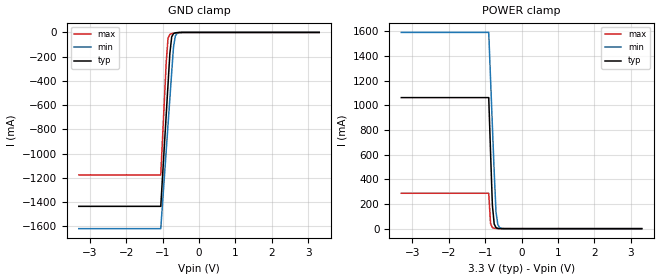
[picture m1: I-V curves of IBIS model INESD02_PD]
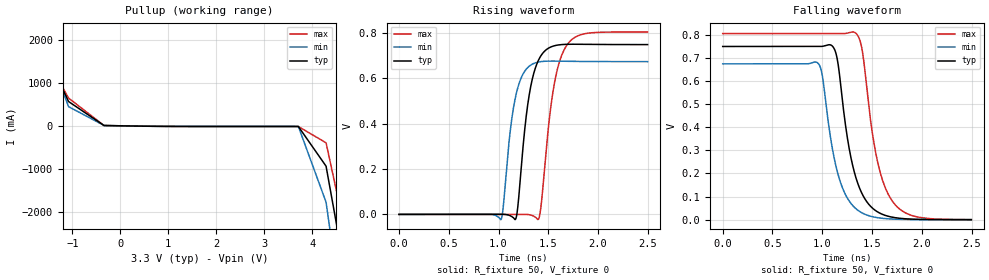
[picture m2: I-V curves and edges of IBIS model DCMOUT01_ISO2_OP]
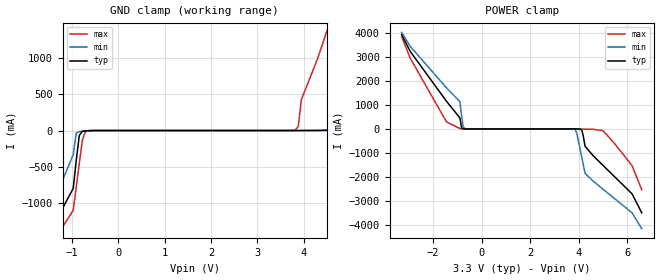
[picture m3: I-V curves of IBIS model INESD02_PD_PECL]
|   This file is an IBIS representation of the   |
|   Integrated Device Technology, Inc.   |
|   ICS841608I   |
|   FEMTOCLOCKS CRYSTAL-TO-HCSL CLOCK GENERATOR   |
[IBIS Ver]   4.1
[File name]   841608i_3v3.ibs
[File Rev]   1.0
[Date]   5 Mar 2010
[Source]   Originated at Integrated Device Technology, Inc.
[Disclaimer]
IDT hereby grants the user of this IBIS model a non-exclusive,
nontransferable license to use this IBIS model under the following terms.
Before using this IBIS model, the user should read this license.
If the user does not accept these terms,  the IBIS model should be
returned to IDT within 30 days.
   The user is granted this license only to use the IBIS model and
is not granted rights to sell, load, rent, lease or license the IBIS
model in whole or in part, or in modified form to anyone other than
user. User may modify the IBIS model to suit its specific
applications but rights to derivative works and such modifications
shall belong to IDT.
   This IBIS model is provided on an "AS IS" basis and IDT makes
absolutely no warranty with respect to the information contained
herein. IDT DISCLAIMS AND CUSTOMER WAIVES ALL WARRANTIES, EXPRESS
OR IMPLIED, INCLUDING WARRANTIES OF MERCHANTABILITY OR FITNESS FOR
A PARTICULAR PURPOSE. The entire risk as to quality and performance
is with the Customer. ACCORDINGLY, IN NO EVENT SHALL THE COMPANY BE
LIABLE FOR ANY DAMAGES, WHETHER IN CONTRACT OR TORT,INCLUDING ANY
LOST PROFITS OR OTHER INCIDENTAL, CONSEQUENTIAL, EXEMPLARY, OR
PUNITIVE DAMAGES ARISING OUT OF THE USE OR APPLICATION OF THE IBIS
model provided in this package. Further, IDT reserves the right to
make changes without notice to any product herein to improve
reliability, function, or design. IDT does not convey any license
under patent rights or any other intellectual property rights,
including those of third parties.
   IDT is not obligated to provide maintenance or support
for the licensed IBIS model.
[Copyright]   Copyright 2008 by Integrated Device Technology, Inc.
[Component]   ICS841608KI
[Manufacturer] Integrated Device Technology, Inc.
[Package]
|LD QFN 32
|lead + wire   typ   min   max
R_pkg   72.4655m   58.886m   86.045m
L_pkg   1.47175nH   1.11650nH   1.77850nH
C_pkg   0.07747pF   0.07444pF   0.08050pF
[Pin] signal_name   model_name   R_pin   L_pin   C_pin
1   XTAL_IN  NC   86.045m   1.77850nH   0.08050pF
2   XTAL_OUT NC   76.996m   1.55783nH   0.07848pF
3   MR/nOE   INESD02_PD   67.941m   1.33717nH   0.07646pF
4   VDD   POWER   58.886m   1.11650nH   0.07444pF
5   Q0   DCMOUT01_ISO2_OP   58.886m   1.11650nH   0.07444pF
6   nQ0   DCMOUT01_ISO2_OP   67.941m   1.33717nH   0.07646pF
7   Q1   DCMOUT01_ISO2_OP   76.996m   1.55783nH   0.07848pF
8   nQ1   DCMOUT01_ISO2_OP   86.045m   1.77850nH   0.08050pF
9   GND   GND   86.045m   1.77850nH   0.08050pF
10   Q2   DCMOUT01_ISO2_OP   76.996m   1.55783nH   0.07848pF
11   nQ2   DCMOUT01_ISO2_OP   67.941m   1.33717nH   0.07646pF
12   Q3   DCMOUT01_ISO2_OP   58.886m   1.11650nH   0.07444pF
13   nQ3   DCMOUT01_ISO2_OP   58.886m   1.11650nH   0.07444pF
14   VDD   POWER   67.941m   1.33717nH   0.07646pF
15   Q4   DCMOUT01_ISO2_OP   76.996m   1.55783nH   0.07848pF
16   nQ4   DCMOUT01_ISO2_OP   86.045m   1.77850nH   0.08050pF
17   Q5   DCMOUT01_ISO2_OP   86.045m   1.77850nH   0.08050pF
18   nQ5   DCMOUT01_ISO2_OP   76.996m   1.55783nH   0.07848pF
19   GDN   GND   67.941m   1.33717nH   0.07646pF
20   Q6   DCMOUT01_ISO2_OP   58.886m   1.11650nH   0.07444pF
21   nQ6   DCMOUT01_ISO2_OP   58.886m   1.11650nH   0.07444pF
22   Q7   DCMOUT01_ISO2_OP   67.941m   1.33717nH   0.07646pF
23   nQ7   DCMOUT01_ISO2_OP   76.996m   1.55783nH   0.07848pF
24   VDD   POWER   86.045m   1.77850nH   0.08050pF
25   FSEL   INESD02_PD   86.045m   1.77850nH   0.08050pF
26   IREF   NC   76.996m   1.55783nH   0.07848pF
27   BYPASS   INESD02_PD   67.941m   1.33717nH   0.07646pF
28   VDDA   POWER   58.886m   1.11650nH   0.07444pF
29   REF_SEL  INESD02_PD   58.886m   1.11650nH   0.07444pF
30   REF_IN   INESD02_PD_PECL   67.941m   1.33717nH   0.07646pF
31   VDD   POWER   76.996m   1.55783nH   0.07848pF
32   GND   GND   86.045m   1.77850nH   0.08050pF
[Diff Pin]  inv_pin  vdiff tdelay_typ tdelay_min  tdelay_max
5   6   NA   0   0   0
7   8   NA   0   0   0
10   11   NA   0   0   0
12   13   NA   0   0   0
15   16   NA   0   0   0
17   18   NA   0   0   0
20   21   NA   0   0   0
22   23   NA   0   0   0
| Models and submodels in the file (3): INESD02_PD (Input), DCMOUT01_ISO2_OP (Open_source), INESD02_PD_PECL (Input)
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[Model]   INESD02_PD
Model_type   Input
Polarity   Non-Inverting
Vinl = 0.80V
Vinh = 2.0V
|   typ   min   max
C_comp   2pF   1.5pF   2.5pF
|   typ   min   max
[Voltage range]  3.3V   3.15V   3.45V
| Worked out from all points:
|   GND clamp passes 1 mA (typ) near -0.56 V on its own axis
|   POWER clamp passes 1 mA (typ) near -0.61 V on its own axis
[GND_clamp]
|Voltage   I(typ)   I(min)   I(max)
-3.3V     -1.436A    -1.62A     -1.176A
-1.05V    -1.436A    -1.62A     -1.176A
-900mV    -678.5mA   -975.1mA   -244mA
-850mV    -426.1mA   -760.1mA   -46.85mA
-800mV    -173.9mA   -545.4mA   -16.11mA
-750mV    -36.96mA   -330.7mA   -9.916mA
-700mV    -9.696mA   -120.2mA   -7.056mA
-650mV    -3.545mA   -29.7mA    -4.857mA
-600mV    -1.629mA   -7.52mA    -3.049mA
-400mV    -52.81uA   -52.52uA   -108.7uA
3.3V      71.13uA    77.43uA    62.11uA
[POWER_clamp]
|Voltage   I(typ)   I(min)   I(max)
-3.3V     1.063A     1.593A     287.3mA
-900mV    1.063A     1.593A     287.3mA
-850mV    620.5mA    1.215A     41.84mA
-800mV    191.6mA    837.5mA    8.757mA
-750mV    37.76mA    460.2mA    3.328mA
-700mV    8.104mA    133.8mA    1.728mA
-650mV    2.076mA    32.66mA    905.3uA
-600mV    678.1uA    8.083mA    443.8uA
-450mV    104.2uA    213.3uA    89.09uA
3.3V      -3.041nA   -3.986uA   0A
[Model]   DCMOUT01_ISO2_OP
Model_type   Open_source
Polarity   Non-Inverting
|   typ   min   max
C_comp   2pF   1.5pF   2.5pF
Vmeas = .344V
Rref = 50
Cref = 0
Vref = 0V
|   typ   min   max
[Voltage range]   3.3V   3.135V   3.465V
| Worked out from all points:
|   slope of the pullup table from 0 to 0.495 V, typ, clamps not added: 54.5 ohm
|   rising waveform, R_fixture 50, V_fixture 0: 20-80 % time 123ps typ, 114ps min, 139ps max; typ from 0 V to 0.749 V
|   falling waveform, R_fixture 50, V_fixture 0: 20-80 % time 182ps typ, 179ps min, 184ps max; typ from 0.749 V to 0 V
[Pullup]
|Voltage   I (typ)   I (min)   I (max)
-3.3V     5.929A     7.281A     5.128A
-2.56V    4.138A     5A         3.631A
-1.82V    2.349A     2.722A     2.136A
-1.08V    565.7mA    446.7mA    647.1mA
-340mV    7.268mA    8.174mA    6.641mA
3.71V     -15.08mA   -14.13mA   -16.17mA
4.288V    -939.9mA   -1.778A    -395.8mA
4.866V    -4.531A    -6.361A    -3.386A
6.6V      -15.32A    -20.11A    -12.39A
[Ramp]
|   typ   min   max
dV/dt_r   0.618/0.195n   0.559/0.181n   0.661/0.221n
dV/dt_f   0.605/0.294n   0.545/0.287n   0.649/0.3n
R_load =   50.0000
[Rising Waveform]
R_fixture = 50
V_fixture = 0
V_fixture_max = 0
V_fixture_min = 0
C_fixture = 0.0p
| Time   typ   min   max
0s        1.469nV    329.3pV    95.28nV
1.026ns   401.4uV    -22.55mV   617.5nV
1.119ns   -5.95mV    370.6mV    -10.36uV
1.171ns   -21.47mV   518.2mV    2.251uV
1.294ns   484.8mV    647.9mV    -448.4uV
1.399ns   677.8mV    671.8mV    -22.17mV
1.429ns   701.6mV    674mV      42.96mV
1.547ns   741.9mV    676.3mV    539.5mV
1.672ns   750mV      675.5mV    736mV
2.498ns   748.9mV    673.8mV    804.6mV
[Falling Waveform]
R_fixture = 50
V_fixture = 0
V_fixture_max = 0
V_fixture_min = 0
C_fixture = 0.0p
| Time   typ   min   max
0s        748.9mV    673.8mV    804.6mV
953.5ps   748.5mV    678.1mV    804.6mV
1.001ns   749.6mV    621.8mV    804.6mV
1.101ns   750.8mV    308.7mV    804.7mV
1.154ns   687.2mV    203.9mV    804.5mV
1.334ns   187.9mV    49.06mV    807.6mV
1.401ns   111mV      28.85mV    732.3mV
1.549ns   35.42mV    9.066mV    263.9mV
1.689ns   12.05mV    3.027mV    89.91mV
2.498ns   24.47uV    5.43uV     200.3uV
[Model]   INESD02_PD_PECL
Model_type  Input
Polarity   Non-Inverting
Vinl = 0.8V
Vinh = 2.0V
|   typ   min   max
C_comp   2pF   1.5pF   2.5pF
|   typ   min   max
[Voltage range]  3.3V   3.15V   3.45V
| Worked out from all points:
|   GND clamp passes 1 mA (typ) near -0.59 V on its own axis
|   POWER clamp passes 1 mA (typ) near -0.70 V on its own axis
[GND_clamp]
-3.3V     -3.894A    -4.294A    -3.674A
-1.6V     -1.569A    -1.322A    -1.74A
-974.8mV  -794.1mA   -331.5mA   -1.096A
-843.4mV  -68.33mA   -15.34mA   -452.9mA
-646.5mV  -1.912mA   -4.151mA   -2.665mA
3.818V    89.38uA    70.49uA    7.198mA
3.95V     342.2uA    75.94uA    423.8mA
4.6V      7.437mA    165.5uA    1.553A
4.9V      78.32mA    440.9uA    2.118A
5.5V      1.293A     2.769mA    3.249A
6.25V     2.651A     112.4mA    4.38A
6.6V      3.331A     896.1mA    4.946A
[POWER_clamp]
-3.3V     3.923A     4.017A     3.838A
-2.95V    3.23A      3.44A      2.951A
-1.45V    1.149A     1.709A     289.6mA
-896.9mV  456.5mA    1.133A     15.4mA
-762.9mV  4.223mA    91.07mA    1.486mA
-695.9mV  792.2uA    10.73mA    555.6uA
3.861V    -556.7uA   -26.14mA   -39.45uA
4.129V    -41.85mA   -1.19A     -4.904mA
4.263V    -724.2mA   -1.847A    -12.04mA
5V        -1.514A    -2.505A    -71.38mA
6.2V      -2.701A    -3.492A    -1.525A
6.6V      -3.492A    -4.151A    -2.536A
